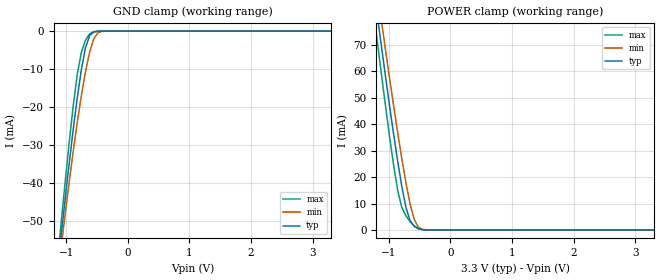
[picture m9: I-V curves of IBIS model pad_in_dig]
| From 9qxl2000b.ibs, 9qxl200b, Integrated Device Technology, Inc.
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|   Model pad_in_dig
[Model] pad_in_dig
Model_type Input
Vinl =   1.00V
Vinh =   2.00V
Polarity   Non-Inverting
C_comp   2.085pF   1.985pF   2.158pF
C_comp_pullup   1.048pF   0.980pF   1.112pF
[Temperature Range]   65.000   0.125k   -10.000
[Voltage Range]   3.300V   3.135V   3.465V
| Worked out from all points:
|   GND clamp passes 1 mA (typ) near -0.61 V on its own axis
|   POWER clamp passes 1 mA (typ) near -0.56 V on its own axis
[GND_clamp]
|Voltage   I(typ)   I(min)   I(max)
-3.3V     -432.5mA   -402.6mA   -464.3mA
-1.089V   -55.08mA   -58.01mA   -51.88mA
-1.022V   -45.08mA   -49.01mA   -40.7mA
-888mV    -26.26mA   -31.97mA   -20.07mA
-821mV    -17.73mA   -24.16mA   -11.52mA
-754mV    -10.22mA   -17.02mA   -5.662mA
-687mV    -4.395mA   -10.74mA   -2.416mA
-620mV    -1.204mA   -5.588mA   -737.3uA
-553mV    -249.8uA   -2.035mA   -151.3uA
-486mV    -49.58uA   -456.4uA   -23.01uA
-352mV    -1.602uA   -12.35uA   -256.1nA
3.3V      0A         0A         0A
[POWER_clamp]
|Voltage   I(typ)   I(min)   I(max)
-3.3V     496.3mA    485.4mA    509mA
-1.256V   94.12mA    102.6mA    85.06mA
-1.189V   82.11mA    91.16mA    72.29mA
-1.122V   70.29mA    79.87mA    59.76mA
-1.055V   58.7mA     68.76mA    47.54mA
-854mV    26.05mA    36.89mA    15.04mA
-787mV    16.5mA     27.04mA    8.511mA
-720mV    8.554mA    17.87mA    5.345mA
-653mV    3.526mA    9.886mA    3.208mA
-586mV    1.393mA    3.993mA    1.561mA
-519mV    483.8uA    1.071mA    518.2uA
3.3V      0A         0A         0A
